| TEXAS INSTRUMENTS INCORPORATED
| Standard Linear and Logic Group
| IBIS Model of SN74AHCT373
| OCTAL TRANSPARENT D-TYPE LATCHES WITH 3-STATE OUTPUTS
| This file contains package information for the following:
|  SSOP 20-pin (DB) package as [Component] AHCT373_DB
|  TVSOP 20-pin (DGV) package as [Component] AHCT373_DGV
|  SOIC 20-pin (DW) package as [Component] AHCT373_DW
|  PDIP 20-pin (N) package as [Component] AHCT373_N
|  TSSOP 20-pin (PW) package as [Component] AHCT373_PW
| This device can be powered at the following Vccs:
|  5 volt Vcc
| This file provides unique models under the [Model Selector] for each Vcc.
| For operation at a specific Vcc, select the appropriate model after each
| [Model Selector] keyword.
[IBIS Ver]   3.2
[Comment char]  |_char
[File Name]   sn74ahct373.ibs
[File Rev]   1.1 | a_die
[Date]   June 11, 2001
[Source]   Data created from TI-SPICE simulations at TI-SLL.
[Notes]   The following is an IBIS list for the AHCT373.
   Please contact sllibis@ti.com with questions and
   comments concerning SLL IBIS models.
   NON MONOTONOCITY IN PULLDOWN DATA
[Disclaimer] Property of Texas Instruments Incorporated.  Unauthorized
   reproduction and/or distribution is strictly prohibited.
   This product is protected under copyright law.
   Created  2001, (C) Copyright  2001, Texas Instruments
   Incorporated, All Rights Reserved
   UNLESS THERE IS A SIGNED, WRITTEN AGREEMENT TO THE
   CONTRARY, TEXAS INSTRUMENTS (TI) IS PROVIDING THE IBIS
   MODELS  AND WITHOUT ANY WARRANTY, EXPRESSED OR
   IMPLIED.  TI assumes no liability for:
   1) the accuracy of the IBIS models provided to your
   company;
   2) the proper functioning of these IBIS Models in your
   design or for any resulting applications; or
   3) infringement of patents, copyrights or intellectual
   property rights resulting from your use of these IBIS
   models.
   TI provides IBIS Models as a service to our customers.
   You and your company shall not distribute, sell or give
   these models to anyone else without prior written
   permission from TI.
   TI reserves the right to make changes to our products or
   to discontinue any semiconductor product or service
   without notice, and advises our customers to obtain the
   latest version of relevant information to verify, before
   placing orders, that the information being relied on is
   current.
   Please be aware that your receipt and use of the IBIS
   information provided shall serve as acceptance of these
   terms and conditions.  If you do not accept these terms,
   you should return or destroy the IBIS models and any
   other accompanying information immediately.
| Component AHCT373_DB 20-pin SSOP
[Component]   AHCT373_DB
[Manufacturer]   Texas Instruments, Inc.
[Package]
|   typ   min   max
R_pkg   4.000e-02   3.500e-02   5.100e-02
L_pkg   3.495e-09   3.035e-09   4.314e-09
C_pkg   4.200e-13   3.460e-13   5.020e-13
[Pin]   signal_name   model_name   R_pin   L_pin   C_pin
1   NOE   AHCT373_OEN   4.900e-02   4.310e-09   5.020e-13
2   1Q   AHCT373_OUT   4.800e-02   3.903e-09   4.870e-13
3   1D   AHCT373_IN   3.500e-02   3.189e-09   3.960e-13
4   2D   AHCT373_IN   3.500e-02   3.036e-09   3.470e-13
5   2Q   AHCT373_OUT   3.500e-02   3.035e-09   3.670e-13
6   3Q   AHCT373_OUT   3.500e-02   3.035e-09   3.670e-13
7   3D   AHCT373_IN   3.500e-02   3.036e-09   3.470e-13
8   4D   AHCT373_IN   3.500e-02   3.189e-09   3.970e-13
9   4Q   AHCT373_OUT   4.700e-02   3.899e-09   4.880e-13
10   GND   GND   5.100e-02   4.314e-09   5.000e-13
11   LE   AHCT373_LE   5.100e-02   4.314e-09   5.000e-13
12   5Q   AHCT373_OUT   4.700e-02   3.899e-09   4.880e-13
13   5D   AHCT373_IN   3.500e-02   3.189e-09   3.970e-13
14   6D   AHCT373_IN   3.500e-02   3.036e-09   3.460e-13
15   6Q   AHCT373_OUT   3.500e-02   3.035e-09   3.670e-13
16   7Q   AHCT373_OUT   3.500e-02   3.035e-09   3.670e-13
17   7D   AHCT373_IN   3.500e-02   3.036e-09   3.460e-13
18   8D   AHCT373_IN   3.500e-02   3.189e-09   3.970e-13
19   8Q   AHCT373_OUT   4.700e-02   3.899e-09   4.880e-13
20   VCC   POWER   5.100e-02   4.314e-09   5.020e-13
| Component AHCT373_DGV 20-pin TVSOP
[Component]   AHCT373_DGV
[Manufacturer]   Texas Instruments, Inc.
[Package]
|   typ   min   max
R_pkg   4.400e-02   3.800e-02   4.800e-02
L_pkg   2.561e-09   2.236e-09   2.961e-09
C_pkg   3.420e-13   2.640e-13   4.460e-13
[Pin]   signal_name   model_name   R_pin   L_pin   C_pin
1   NOE   AHCT373_OEN   4.400e-02   2.935e-09   4.170e-13
2   1Q   AHCT373_OUT   4.200e-02   2.869e-09   4.460e-13
3   1D   AHCT373_IN   4.300e-02   2.399e-09   3.160e-13
4   2D   AHCT373_IN   4.400e-02   2.236e-09   2.650e-13
5   2Q   AHCT373_OUT   4.600e-02   2.278e-09   2.640e-13
6   3Q   AHCT373_OUT   4.500e-02   2.274e-09   2.640e-13
7   3D   AHCT373_IN   4.400e-02   2.285e-09   2.690e-13
8   4D   AHCT373_IN   4.300e-02   2.452e-09   3.200e-13
9   4Q   AHCT373_OUT   4.400e-02   2.900e-09   4.460e-13
10   GND   GND   4.400e-02   2.961e-09   4.180e-13
11   LE   AHCT373_LE   4.500e-02   2.954e-09   4.180e-13
12   5Q   AHCT373_OUT   4.200e-02   2.847e-09   4.430e-13
13   5D   AHCT373_IN   4.500e-02   2.453e-09   3.190e-13
14   6D   AHCT373_IN   4.500e-02   2.297e-09   2.690e-13
15   6Q   AHCT373_OUT   4.800e-02   2.334e-09   2.680e-13
16   7Q   AHCT373_OUT   4.800e-02   2.335e-09   2.670e-13
17   7D   AHCT373_IN   4.600e-02   2.299e-09   2.680e-13
18   8D   AHCT373_IN   4.600e-02   2.457e-09   3.200e-13
19   8Q   AHCT373_OUT   4.300e-02   2.848e-09   4.410e-13
20   VCC   POWER   3.800e-02   2.812e-09   4.080e-13
| Component AHCT373_DW 20-pin SOIC
[Component]   AHCT373_DW
[Manufacturer]   Texas Instruments, Inc.
[Package]
|   typ   min   max
R_pkg   3.800e-02   3.300e-02   4.500e-02
L_pkg   5.012e-09   4.110e-09   6.349e-09
C_pkg   7.170e-13   5.300e-13   8.680e-13
[Pin]   signal_name   model_name   R_pin   L_pin   C_pin
1   NOE   AHCT373_OEN   4.200e-02   6.336e-09   8.650e-13
2   1Q   AHCT373_OUT   4.300e-02   5.542e-09   8.670e-13
3   1D   AHCT373_IN   3.400e-02   4.714e-09   7.320e-13
4   2D   AHCT373_IN   3.400e-02   4.377e-09   5.910e-13
5   2Q   AHCT373_OUT   3.600e-02   4.130e-09   5.330e-13
6   3Q   AHCT373_OUT   3.500e-02   4.111e-09   5.300e-13
7   3D   AHCT373_IN   3.400e-02   4.284e-09   5.830e-13
8   4D   AHCT373_IN   3.400e-02   4.634e-09   7.260e-13
9   4Q   AHCT373_OUT   4.000e-02   5.518e-09   8.650e-13
10   GND   GND   4.300e-02   6.349e-09   8.660e-13
11   LE   AHCT373_LE   4.100e-02   6.281e-09   8.610e-13
12   5Q   AHCT373_OUT   4.500e-02   5.561e-09   8.680e-13
13   5D   AHCT373_IN   3.300e-02   4.778e-09   7.420e-13
14   6D   AHCT373_IN   3.500e-02   4.414e-09   5.960e-13
15   6Q   AHCT373_OUT   3.500e-02   4.110e-09   5.330e-13
16   7Q   AHCT373_OUT   3.600e-02   4.130e-09   5.330e-13
17   7D   AHCT373_IN   3.400e-02   4.377e-09   5.910e-13
18   8D   AHCT373_IN   3.400e-02   4.714e-09   7.310e-13
19   8Q   AHCT373_OUT   4.300e-02   5.569e-09   8.680e-13
20   VCC   POWER   4.200e-02   6.308e-09   8.640e-13
| Component AHCT373_N 20-pin PDIP
[Component]   AHCT373_N
[Manufacturer]   Texas Instruments, Inc.
[Package]
|   typ   min   max
R_pkg   4.300e-02   3.800e-02   5.000e-02
L_pkg   7.384e-09   4.680e-09   1.032e-08
C_pkg   5.100e-13   2.310e-13   8.210e-13
[Pin]   signal_name   model_name   R_pin   L_pin   C_pin
1   NOE   AHCT373_OEN   4.200e-02   9.427e-09   8.100e-13
2   1Q   AHCT373_OUT   4.600e-02   8.544e-09   4.560e-13
3   1D   AHCT373_IN   4.800e-02   7.163e-09   4.350e-13
4   2D   AHCT373_IN   4.000e-02   4.825e-09   2.610e-13
5   2Q   AHCT373_OUT   4.000e-02   5.284e-09   6.480e-13
6   3Q   AHCT373_OUT   4.000e-02   4.686e-09   2.320e-13
7   3D   AHCT373_IN   4.000e-02   6.359e-09   4.890e-13
8   4D   AHCT373_IN   3.800e-02   7.982e-09   4.750e-13
9   4Q   AHCT373_OUT   4.300e-02   9.403e-09   4.750e-13
10   GND   GND   5.000e-02   1.032e-08   8.050e-13
11   LE   AHCT373_LE   5.000e-02   1.028e-08   8.100e-13
12   5Q   AHCT373_OUT   4.300e-02   9.383e-09   4.770e-13
13   5D   AHCT373_IN   3.800e-02   7.978e-09   4.760e-13
14   6D   AHCT373_IN   4.000e-02   6.302e-09   4.920e-13
15   6Q   AHCT373_OUT   4.000e-02   4.680e-09   2.310e-13
16   7Q   AHCT373_OUT   4.000e-02   5.284e-09   6.480e-13
17   7D   AHCT373_IN   4.000e-02   4.822e-09   2.610e-13
18   8D   AHCT373_IN   4.700e-02   7.118e-09   4.390e-13
19   8Q   AHCT373_OUT   4.600e-02   8.492e-09   4.610e-13
20   VCC   POWER   4.300e-02   9.348e-09   8.210e-13
| Component AHCT373_PW 20-pin TSSOP
[Component]   AHCT373_PW
[Manufacturer]   Texas Instruments, Inc.
[Package]
|   typ   min   max
R_pkg   4.500e-02   3.600e-02   5.700e-02
L_pkg   2.694e-09   2.290e-09   3.177e-09
C_pkg   1.560e-13   7.600e-14   2.590e-13
[Pin]   signal_name   model_name   R_pin   L_pin   C_pin
1   NOE   AHCT373_OEN   3.600e-02   3.045e-09   2.590e-13
2   1Q   AHCT373_OUT   5.100e-02   3.013e-09   1.890e-13
3   1D   AHCT373_IN   4.400e-02   2.695e-09   1.640e-13
4   2D   AHCT373_IN   4.700e-02   2.362e-09   7.900e-14
5   2Q   AHCT373_OUT   4.700e-02   2.333e-09   8.600e-14
6   3Q   AHCT373_OUT   4.700e-02   2.298e-09   8.500e-14
7   3D   AHCT373_IN   4.700e-02   2.351e-09   7.900e-14
8   4D   AHCT373_IN   4.400e-02   2.706e-09   1.650e-13
9   4Q   AHCT373_OUT   4.900e-02   2.999e-09   1.880e-13
10   GND   GND   3.900e-02   3.039e-09   2.570e-13
11   LE   AHCT373_LE   3.800e-02   3.044e-09   2.580e-13
12   5Q   AHCT373_OUT   5.700e-02   3.177e-09   1.990e-13
13   5D   AHCT373_IN   4.400e-02   2.825e-09   1.730e-13
14   6D   AHCT373_IN   4.700e-02   2.429e-09   8.300e-14
15   6Q   AHCT373_OUT   4.900e-02   2.383e-09   9.000e-14
16   7Q   AHCT373_OUT   4.900e-02   2.347e-09   8.900e-14
17   7D   AHCT373_IN   4.700e-02   2.290e-09   7.600e-14
18   8D   AHCT373_IN   4.500e-02   2.613e-09   1.580e-13
19   8Q   AHCT373_OUT   4.400e-02   2.883e-09   1.810e-13
20   VCC   POWER   3.900e-02   3.044e-09   2.560e-13
| Models and submodels in the file (4): AHCT373_IN (Input), AHCT373_OEN (Input), AHCT373_LE (Input), AHCT373_OUT (3-state)
